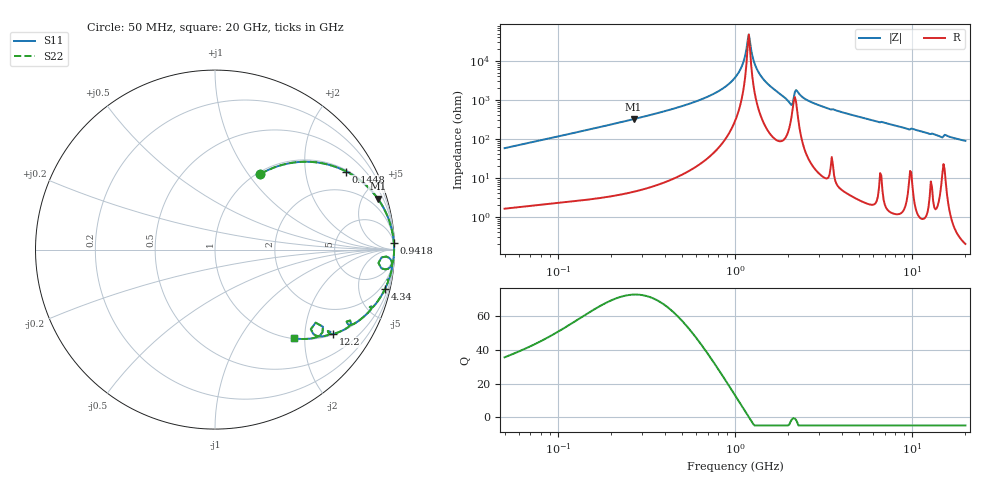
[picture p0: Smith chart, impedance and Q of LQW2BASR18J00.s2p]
!Murata Part Number: LQW2BASR18J00
!These Parameters are Measured in Series Mode Connection
!  o--[Z]--o
!Port1  Port2
!  o-------o
!Freq. Start=50[MHz] Stop=20[GHz], 401[Steps]
# Hz S RI R 50
!Freq.(Hz) S11(Real) S11(Imag) S21(Real) S21(Imag) S12(Real) S12(Imag) S22(Real) S22(Imag)
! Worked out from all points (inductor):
!   401 points, 50 MHz to 20 GHz, reference 50 ohm
!   read as one part in series: L = 182 nH near 51.52 MHz
!   highest Q = 73 at 267.6 MHz (marker M1), where L = 189 nH
!   self-resonance near 1.179 GHz
!   S11 on the Smith chart (normalised r, x): 50 MHz: 1.03, +1.15; 144.8 MHz: 1.05, +3.33; 941.8 MHz: 4, +55; 4.34 GHz: 1.08, -8.70; 12.2 GHz: 1.03, -2.79; 20 GHz: 1.00, -1.76
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5e7  0.2534 0.4211  0.7466 -0.4211  0.7466 -0.4211  0.2534 0.4211
1.364002e8  0.7073 0.4467  0.2927 -0.4467  0.2927 -0.4467  0.7073 0.4467
1.448224e8  0.7316 0.435  0.2684 -0.435  0.2684 -0.435  0.7316 0.435
2.676374e8  0.907 0.2837  0.093 -0.2837  0.093 -0.2837  0.907 0.2837
3.721004e8  0.9531 0.2044  0.0469 -0.2044  0.0469 -0.2044  0.9531 0.2044
6.774326e8  0.9899 0.0882  0.0101 -0.0882  0.0101 -0.0882  0.9899 0.0882
9.418449e8  0.9966 0.036  0.00338 -0.036  0.00338 -0.036  0.9966 0.036
1e9  0.9972 0.0269  0.0028 -0.0269  0.0028 -0.0269  0.9972 0.0269
1.094034e9  0.9977 0.0134  0.00226 -0.0134  0.00226 -0.0134  0.9977 0.0134
1.161586e9  0.9979 0.0044  0.00212 -0.0044  0.00212 -0.0044  0.9979 0.0044
1.196911e9  0.9979 -0.000125  0.00211 0.000125  0.00211 0.000125  0.9979 -0.000125
1.214974e9  0.9979 -0.00239  0.00212 0.00239  0.00212 0.00239  0.9979 -0.00239
1.270815e9  0.9978 -0.00924  0.00223 0.00924  0.00223 0.00924  0.9978 -0.00924
1.329223e9  0.9975 -0.0162  0.00245 0.0162  0.00245 0.0162  0.9975 -0.0162
1.544007e9  0.9958 -0.0403  0.00416 0.0403  0.00416 0.0403  0.9958 -0.0403
2.05233e9  0.9488 -0.1105  0.0512 0.1105  0.0512 0.1105  0.9488 -0.1105
2.245319e9  0.9787 -0.055  0.0213 0.055  0.0213 0.055  0.9787 -0.055
2.728004e9  0.9835 -0.1156  0.0165 0.1156  0.0165 0.1156  0.9835 -0.1156
4.34015e9  0.9481 -0.2176  0.0519 0.2176  0.0519 0.2176  0.9481 -0.2176
7.442007e9  0.8478 -0.3564  0.1522 0.3564  0.1522 0.3564  0.8478 -0.3564
1.220001e10  0.6594 -0.4694  0.3406 0.4694  0.3406 0.4694  0.6594 -0.4694
2e10  0.4377 -0.495  0.5623 0.495  0.5623 0.495  0.4377 -0.495
